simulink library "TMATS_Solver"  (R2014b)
settings: Solver=ode45  StartTime=0.0  StopTime=10.0  RelTol=1e-3
libraries: Lib_Solve_DataOut_TMATS x1, Lib_Solve_IterNRSolverJC_TMATS x1, Lib_Solve_ModelSource_TMATS x1, Lib_Solve_OuterLoopIntegrator_TMATS x1, Lib_Solve_ParameterRamp_TMATS x1, Lib_Solve_ParameterStep_TMATS x1, Lib_Solve_SSNRSolverJC_TMATS x1, Lib_Solve_VectorCondition_TMATS x1

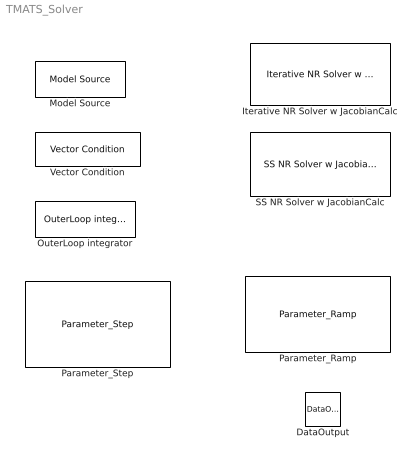
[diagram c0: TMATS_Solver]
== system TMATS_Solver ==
  DataOutput : Lib_Solve_DataOut_TMATS/DataOutput  Var_M='Scalar'  SVar_M=gcb
  Iterative NR Solver w JacobianCalc : Lib_Solve_IterNRSolverJC_TMATS/Iterative NR Solver w JacobianCalc  SJac_Per_M=[0.01; 0.05; 0.05]  SNR_IC_M=[1; 2; 3]  SNR_DX_M=5  SJacobianAttempts_M=20  Cond_Limits_M=0.01
  Model Source : Lib_Solve_ModelSource_TMATS/Model Source  T_vec_M=[0 5 10 100]  input_array_M=[10000 10000 12000 12000]
  OuterLoop integrator : Lib_Solve_OuterLoopIntegrator_TMATS/OuterLoop integrator  OL_IC_M=10000
  Parameter_Ramp : Lib_Solve_ParameterRamp_TMATS/Parameter_Ramp  BN_M='Testing_Output/Subsystem1'  PN_M='Test_M'  IV_M='[1]'  FV_M='[5]'  ST_M=3  ET_M=6
  Parameter_Step : Lib_Solve_ParameterStep_TMATS/Parameter_Step  BN_M='Testing_Output/Subsystem1'  PN_M='Test_M'  IV_M='[3 4; 5 6]'  FV_M='[5 6; 3 4]'  ST_M=3
  SS NR Solver w JacobianCalc : Lib_Solve_SSNRSolverJC_TMATS/SS NR Solver w JacobianCalc  SJac_Per_M=[0.01; 0.05; 0.05]  SNR_IC_M=[1; 2; 3]  SNR_DX_M=5  SJacobianAttempts_M=20  Cond_Limits_M=0.1
  Vector Condition : Lib_Solve_VectorCondition_TMATS/Vector Condition  Cond_Limits_M=0.01
